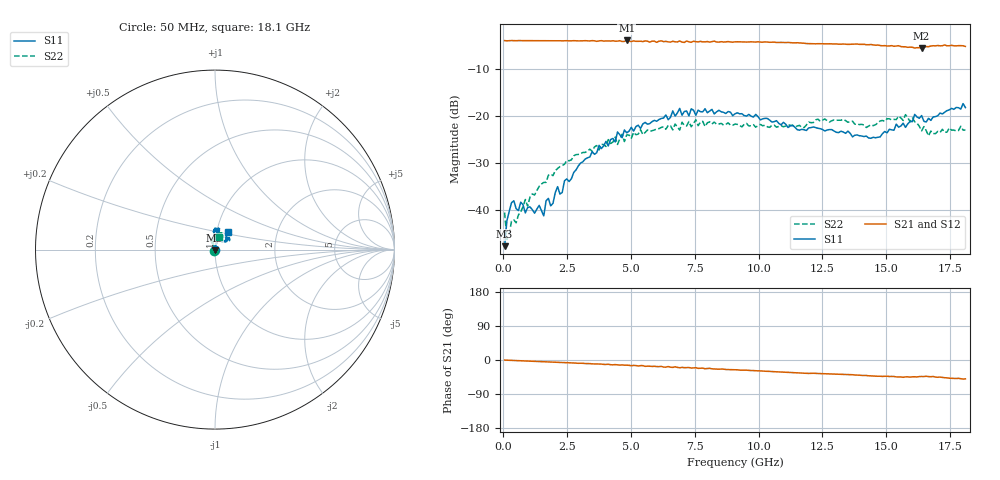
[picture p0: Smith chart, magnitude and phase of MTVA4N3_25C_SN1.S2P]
! Network Analyzer HP8720D.06.14 Serial No. US36140669
! 11 May 2005  09:46:54
! Frequency  S11  S21  S12  S22
# HZ  S  DB R 50
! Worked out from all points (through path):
!   201 points, 50 MHz to 18.1 GHz, reference 50 ohm
!   highest |S21| = -3.83 dB at 4.833 GHz (marker M1); lowest = -5.5 dB at 16.39 GHz (marker M2)
!   group delay of S21, straight-line fit = 7.72 ps
!   lowest |S11| = -47.7 dB at 50 MHz (marker M3), VSWR 1.01, Z = 49.7 - j0.303 ohm
!   |S11| at or under -10 dB: start of sweep to end of sweep
!   |S22| runs from -46.3 to -19.7 dB; largest |S21 - S12| = 0.024
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5e7  -47.72 -132.1  -3.86 -0.2  -3.90 -0.6  -40.54 -142.8
1.4025e8  -42.27 -160.8  -3.91 -0.5  -3.90 -0.9  -46.30 -173.7
3.2075e8  -38.45 -179.1  -3.85 -0.9  -3.87 -1.3  -42.39 -174.6
5.0125e8  -39.69 -171.6  -3.89 -1.6  -3.87 -1.9  -42.73 152.7
8.6225e8  -40.62 161.1  -3.87 -2.5  -3.89 -2.9  -37.76 147.2
1.40375e9  -39.02 137.7  -3.88 -4.1  -3.89 -4.5  -34.97 128.0
1.58425e9  -41.25 117.7  -3.90 -4.7  -3.89 -5.0  -34.11 120.6
1.6745e9  -38.04 108.9  -3.88 -4.8  -3.89 -5.2  -34.11 121.1
1.855e9  -39.12 117.5  -3.90 -5.4  -3.89 -5.7  -32.37 115.3
2.12575e9  -35.02 99.6  -3.89 -6.2  -3.89 -6.5  -31.15 111.3
2.30625e9  -36.27 83.9  -3.92 -6.6  -3.90 -6.9  -30.48 110.8
3.1185e9  -29.70 77.4  -3.91 -8.8  -3.93 -9.4  -27.74 119.7
4.83325e9  -23.53 81.0  -3.83 -13.6  -3.91 -14.7  -23.99 94.5
6.09675e9  -20.70 80.0  -3.99 -17.4  -3.93 -17.7  -22.64 88.2
6.909e9  -18.33 81.2  -3.94 -20.4  -4.06 -19.9  -22.93 79.7
9.075e9  -19.48 90.5  -4.13 -25.8  -4.09 -26.2  -21.67 70.7
1.21435e10  -22.28 90.1  -4.53 -35.0  -4.50 -35.5  -21.35 76.5
1.439975e10  -24.70 45.8  -4.69 -42.0  -4.67 -42.2  -21.83 75.3
1.512175e10  -22.78 40.6  -5.00 -43.6  -4.87 -43.6  -20.55 75.1
1.57535e10  -22.37 40.5  -5.18 -44.5  -5.34 -45.7  -19.65 65.9
1.638525e10  -19.85 35.4  -5.47 -43.5  -5.30 -43.4  -23.11 59.0
1.81e10  -18.15 54.2  -5.11 -49.8  -5.14 -51.0  -22.94 71.1
